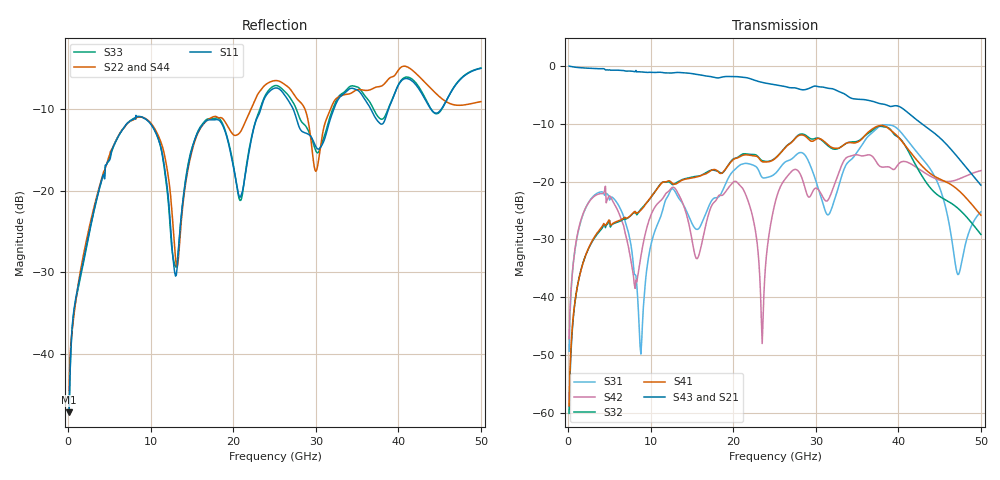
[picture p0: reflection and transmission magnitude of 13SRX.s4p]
! DAC39RF10ACK
! 256-pin FCBGA package
! Texas Instruments 8/20/2022
! Single-ended  S-parameters
! PORT#  PORT_NAME  NET_NAME
! PORT1:  xSRXN.DIEBUMP  xSRXN
! PORT2:  xSRXN.BGA  xSRXN
! PORT3:  xSRXP.DIEBUMP  xSRXP
! PORT4:  xSRXP.BGA  xSRXP
! Touchstone Ver. 1.0
! Number of ports is 4
# Hz	S	MA	R	50.000000
! SCATTERING PARAMETERS  :
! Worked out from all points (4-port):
!   500 points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, 100 MHz to 50 GHz, reference 50 ohm
!   strongest paths, dB at 100 MHz, 12.6 GHz, 25.1 GHz, 37.6 GHz, 50 GHz:
!     S43: 0.0, -1.2, -3.3, -6.4, -20.6
!     S21: 0.0, -1.2, -3.3, -6.3, -20.5
!     S41: -58.8, -20.3, -16.0, -10.4, -25.8
!     S32: -60.1, -20.5, -15.9, -10.4, -29.1
!     S42: -47.2, -21.0, -23.4, -17.1, -18.1
!     S31: -49.3, -21.2, -18.6, -10.6, -25.2
!   lowest |S11| = -47.1 dB at 100 MHz (marker M1), VSWR 1.01, Z = 50.4 + j0.24 ohm
!   |S11| at or under -10 dB: start of sweep to 23.34 GHz; 27.23 GHz to 32.2 GHz (4.97 GHz wide, 16.7 % of centre); 36.64 GHz to 38.83 GHz (2.19 GHz wide, 5.8 % of centre)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
1e8  0.004434 32.5  0.9916 -2.8  0.003399 84.6  0.001036 -102.9
     0.9959 -2.5  0.00604 33.5  0.001148 -99.4  0.004473 73.7
     0.00341 84.5  0.0009914 -100.1  0.00436 31.4  0.9907 -2.8
     0.001148 -99.4  0.004385 76.5  0.9959 -2.5  0.00622 32.2
2.8e9  0.06444 32.0  0.9506 -64.4  0.07162 21.5  0.02946 -165.8
       0.9528 -64.2  0.06796 -6.7  0.02974 -165.0  0.07097 24.1
       0.07163 21.6  0.02942 -165.7  0.06337 32.0  0.9508 -64.4
       0.02987 -165.0  0.07078 24.3  0.953 -64.2  0.06721 -7.2
7.7e9  0.2699 -71.4  0.8912 -173.7  0.02526 -95.5  0.05154 87.0
       0.8985 -173.7  0.2681 -98.4  0.05181 86.9  0.0181 -122.8
       0.02512 -97.5  0.0519 86.8  0.2713 -71.9  0.8929 -173.9
       0.05224 87.1  0.01871 -124.2  0.901 -173.6  0.2706 -98.3
1.57e10  0.2267 -85.3  0.8437 7.3  0.0384 172.1  0.1097 -89.6
         0.8451 7.5  0.2241 -87.3  0.1107 -89.7  0.02119 30.7
         0.03872 171.1  0.1113 -90.0  0.2296 -84.2  0.8414 7.4
         0.1104 -89.8  0.02193 32.1  0.843 7.5  0.2262 -88.6
2.37e10  0.3589 -56.5  0.7173 -173.4  0.106 -145.3  0.1464 85.6
         0.7197 -173.2  0.4336 -117.3  0.1494 85.0  0.00935 127.0
         0.1073 -145.1  0.1503 84.9  0.3657 -56.7  0.7134 -173.3
         0.1477 85.6  0.01041 125.2  0.7152 -173.4  0.4334 -118.0
3.15e10  0.2472 -84.5  0.6364 13.7  0.05144 177.1  0.2073 -107.1
         0.6359 13.6  0.2906 -116.3  0.2025 -108.7  0.06767 -171.3
         0.05158 177.3  0.2031 -108.8  0.2594 -85.5  0.6461 11.7
         0.2071 -107.2  0.06965 -171.7  0.641 12.1  0.2908 -114.9
5e10  0.5578 -124.9  0.07973 -9.3  0.05422 134.8  0.03589 -162.8
      0.09456 -12.6  0.3494 -162.5  0.04409 -168.2  0.1225 53.5
      0.05477 139.1  0.03493 -159.7  0.56 -126.4  0.08186 -7.8
      0.05117 -170.8  0.1244 52.4  0.09314 -13.6  0.3474 -161.6
